| DDR2_v3p3_1p8v_bd\b17a_v5p0_1p8v_bd.ibs * IBIS 5.0 Model
| Die rev "A"
| 512Gb High Speed TLC Nand Flash IBIS Model
| VCC=2.7V-3.6V, VCCQ=1.7V-1.95V
| Temperature range, Commercial 0C to 70C.
| Part Number   VCC/VCCQ   Architecture  Mode   Package
| MT29F512G08EBCAFB17A  3.3/1.8V   512Gig x 8   NV-DDR2  Bare Die
[IBIS Ver]   5.0
[File name]   DDR2_v3p3_1p8v_bd.ibs
[Date]   01/31/2018
[File Rev]   2.0
[Source]   From silicon level SPICE model at Micron Technology, Inc.
   For support e-mail modelsupport@micron.com
[Notes]   Revision History:
   Rev 1.0: 12/12/2016
   - First revision pre-silicon model from parasitic extracted netlist
   Rev 2.0: 01/31/2018
   - Matched C_comp with latest IOCAP measurements
   - Matched IV curves with latest silicon measurements
   Notes:
   - This IBIS file uses the Submodel keyword to model the
   NV-DDR2 On-die Termination(ODT) characteristics.
   - The C_comp value in the DQ model is set to match the input
   state of the DQ I/O as measured from the HSpice model.
   Due to the C_comp differences between the DQ model and the
   DQ_ODT* models, the output characteristics of the
   models will look different when simulated. To match most
   closely with the HSPICE model, simulate with the
   DQ_35 or DQ_50 model for ALL Output simulations.
   Use the ODT models ONLY for Input simulations.
   - All Submodels: when running through ibischk4.2, this file
   contains warnings about GND and Power Clamp data being
   non-monotonic. When Submodel I-V curves are added to
   non-ODT Power and GND Clamp curves, the resultant
   curve is monotonic. This is not checked correctly with this
   version of the IBIS parser.
   - No Power Clamp Diode in models INPUT, CE_INPUT, WP_INPUT
   and RDBY
   - Typ and slow corner V-t curves in the DQ* models
   are shifted relative to strong corner V-t curve
   to contain all 3 corners within appropriate V-t window
   Models   Typ   Slow   V-t duration
   DQ_35_EXT_ZQ  -0.16ns   -0.39ns   2.38ns
   DQ_50_EXT_ZQ  -0.16ns   -0.39ns   2.38ns
   DQ_35_NO_ZQ   -0.16ns   -0.39ns   2.38ns
   DQ_50_NO_ZQ   -0.16ns   -0.39ns   2.38ns
   - Due to the shift in typ and slow corner, the V-t curves
   may overlap each other. This does not effect the accuracy
   of the IBIS data.
   - Model syntax should be checked using the latest IBISCHK parser,
   Version 6.1.2 or later.  Earlier versions may indicate erroneous
   Errors, Warnings or Cautions due to parser bugs.
   - All DQ/DQS models require overclocking due to inclusion of
   Composite Current data.
   - IBIS Quality Specification 2.0 Summary:
   IQ Score: IQ3MSX
   See Micron IBIS Model Quality Report and Quality Checklist
   for full IQ details
[Disclaimer]  This software code and all associated documentation, comments
   or other information (collectively "Software") is provided
   "AS IS" without warranty of any kind. MICRON TECHNOLOGY, INC.
   ("MTI") EXPRESSLY DISCLAIMS ALL WARRANTIES EXPRESS OR IMPLIED,
   INCLUDING BUT NOT LIMITED TO, NONINFRINGEMENT OF THIRD PARTY
   RIGHTS, AND ANY IMPLIED WARRANTIES OF MERCHANTABILITY OR
   FITNESS FOR ANY PARTICULAR PURPOSE. MTI DOES NOT WARRANT THAT
   THE SOFTWARE WILL MEET YOUR REQUIREMENTS, OR THAT THE
   OPERATION OF THE SOFTWARE WILL BE UNINTERRUPTED OR ERROR-FREE.
   FURTHERMORE, MTI DOES NOT MAKE ANY REPRESENTATIONS REGARDING
   THE USE OR THE RESULTS OF THE USE OF THE SOFTWARE IN TERMS OF
   ITS CORRECTNESS, ACCURACY, RELIABILITY, OR OTHERWISE. THE
   ENTIRE RISK ARISING OUT OF USE OR PERFORMANCE OF THE SOFTWARE
   REMAINS WITH YOU. IN NO EVENT SHALL MTI, ITS AFFILIATED
   COMPANIES OR THEIR SUPPLIERS BE LIABLE FOR ANY DIRECT,
   INDIRECT, CONSEQUENTIAL, INCIDENTAL, OR SPECIAL DAMAGES
   (INCLUDING, WITHOUT LIMITATION, DAMAGES FOR LOSS OF PROFITS,
   BUSINESS INTERRUPTION, OR LOSS OF INFORMATION) ARISING OUT OF
   YOUR USE OF OR INABILITY TO USE THE SOFTWARE, EVEN IF MTI HAS
   BEEN ADVISED OF THE POSSIBILITY OF SUCH DAMAGES. Because some
   jurisdictions prohibit the exclusion or limitation of
   liability for consequential or incidental damages, the above
   limitation may not apply to you.
[Copyright]   Copyright 2018 Micron Technology, Inc. All rights reserved.
|   COMPONENT: MT29F512G08EBCAFB17A
[Component]   MT29F512G08EBCAFB17A
[Manufacturer]  Micron Technology, Inc.
[Package]
| variable   typ   min   max
R_pkg   0.001m   0.001m   0.001m
L_pkg   0.001nH   0.001nH   0.001nH
C_pkg   0.001pf   0.001pf   0.001pf
[Pin]   signal_name model_name   R_pin   L_pin   C_pin
1   VSS   GND
2   VSS   GND
3   VCC   POWER
4   DNU   NC
5   MDS3   NC
6   MDS2   NC
7   MDS1   NC
8   MDS0   NC
9   Eno   NC
10   Eni   NC
11   WP#   WP_INPUT
12   DNU   NC
13   ALE   INPUT
14   CLE   INPUT
15   VSS   GND
16   VCC   POWER
17   VCCQ   POWER
18   DQ0   DQ
19   DQ1   DQ
20   VSSQ   GND
21   DQ2   DQ
22   DQ3   DQ
23   VCCQ   POWER
24   DQS_c   DQS
25   DQS_t   DQS
26   VSSQ   GND
27   DQ4   DQ
28   DQ5   DQ
29   VCCQ   POWER
30   DQ6   DQ
31   DQ7   DQ
32   VSSQ   GND
33   RE_c   RE
34   RE_t   RE
35   VCCQ   POWER
36   VCC   POWER
37   WE#   INPUT
38   DNU   NC
39   CE#   CE_INPUT
40   DNU   NC
41   RB#   RDBY
42   VCCQ   POWER
43   VREFQ   POWER
44   VSSQ   GND
45   ZQ   NC
46   VCCQ   POWER
47   VPP   POWER
48   DNU   NC
49   DNU   NC
50   VCC   POWER
|**********************DIFF PIN*********************************************
[Diff_pin]   inv_pin   vdiff   tdelay_typ   tdelay_min   tdelay_max
   25   24   0.300V   0ns   NA   NA
   34   33   0.300V   0ns   NA   NA
|   Model Selector
[Model Selector] DQ
DQ_35_EXT_ZQ   35 Ohm Data I/O with no ODT, With ZQ Cal
DQ_50_EXT_ZQ   50 Ohm Data I/O with no ODT, With ZQ Cal
DQ_IN_ODT50_EXT_ZQ   Data Input with 50ohm ODT, With ZQ Cal
DQ_IN_ODT75_EXT_ZQ   Data Input with 75ohm ODT, With ZQ Cal
DQ_IN_ODT100_EXT_ZQ   Data Input with 100ohm ODT, With ZQ Cal
DQ_IN_ODT150_EXT_ZQ   Data Input with 150ohm ODT, With ZQ Cal
DQ_25_NO_ZQ   25 Ohm Data I/O with no ODT, With No Cal
DQ_35_NO_ZQ   35 Ohm Data I/O with no ODT, With No Cal
DQ_50_NO_ZQ   50 Ohm Data I/O with no ODT, With No Cal
DQ_IN_ODT50_NO_ZQ   Data Input with 50ohm ODT, With No Cal
DQ_IN_ODT75_NO_ZQ   Data Input with 75ohm ODT, With No Cal
DQ_IN_ODT100_NO_ZQ   Data Input with 100ohm ODT, With No Cal
DQ_IN_ODT150_NO_ZQ   Data Input with 150ohm ODT, With No Cal
[Model Selector] DQS
DQS_35_EXT_ZQ   35 Ohm Data Strobe I/O with no ODT, With ZQ Cal
DQS_50_EXT_ZQ   50 Ohm Data Strobe I/O with no ODT, With ZQ Cal
DQS_IN_ODT50_EXT_ZQ   Data Strobe Input with 50ohm ODT, With ZQ Cal
DQS_IN_ODT75_EXT_ZQ   Data Strobe Input with 75ohm ODT, With ZQ Cal
DQS_IN_ODT100_EXT_ZQ   Data Strobe Input with 100ohm ODT, With ZQ Cal
DQS_IN_ODT150_EXT_ZQ   Data Strobe Input with 150ohm ODT, With ZQ Cal
DQS_25_NO_ZQ   25 Ohm Data Strobe I/O with no ODT, With No Cal
DQS_35_NO_ZQ   35 Ohm Data Strobe I/O with no ODT, With No Cal
DQS_50_NO_ZQ   50 Ohm Data Strobe I/O with no ODT, With No Cal
DQS_IN_ODT50_NO_ZQ   Data Strobe Input with 50ohm ODT, With No Cal
DQS_IN_ODT75_NO_ZQ   Data Strobe Input with 75ohm ODT, With No Cal
DQS_IN_ODT100_NO_ZQ   Data Strobe Input with 100ohm ODT, With No Cal
DQS_IN_ODT150_NO_ZQ   Data Strobe Input with 150ohm ODT, With No Cal
[Model Selector] RE
RE_INPUT   RE Input Model with no ODT
RE_INPUT_ODT50_EXT_ZQ   RE Input Model with 50ohm ODT, With ZQ Cal
RE_INPUT_ODT75_EXT_ZQ   RE Input Model with 75ohm ODT, With ZQ Cal
RE_INPUT_ODT100_EXT_ZQ  RE Input Model with 100ohm ODT, With ZQ Cal
RE_INPUT_ODT150_EXT_ZQ  RE Input Model with 150ohm ODT, With ZQ Cal
RE_INPUT_ODT50_NO_ZQ   RE Input Model with 50ohm ODT, With No Cal
RE_INPUT_ODT75_NO_ZQ   RE Input Model with 75ohm ODT, With No Cal
RE_INPUT_ODT100_NO_ZQ   RE Input Model with 100ohm ODT, With No Cal
RE_INPUT_ODT150_NO_ZQ   RE Input Model with 150ohm ODT, With No Cal
[Model Selector] RDBY
RDBY_FULL   FULL-Drv RDBY Open-Drain Model
RDBY_3QTR   3QTR-Drv RDBY Open-Drain Model
RDBY_HALF   HALF-Drv RDBY Open-Drain Model
RDBY_QTR   QTR-Drv RDBY Open-Drain Model
| Models and submodels in the file (50): DQ_35_EXT_ZQ (I/O), DQ_50_EXT_ZQ (I/O), DQ_IN_ODT50_EXT_ZQ (Input), DQ_IN_ODT75_EXT_ZQ (Input), DQ_IN_ODT100_EXT_ZQ (Input), DQ_IN_ODT150_EXT_ZQ (Input), DQ_25_NO_ZQ (I/O), DQ_35_NO_ZQ (I/O), DQ_50_NO_ZQ (I/O), DQ_IN_ODT50_NO_ZQ (Input), DQ_IN_ODT75_NO_ZQ (Input), DQ_IN_ODT100_NO_ZQ (Input), DQ_IN_ODT150_NO_ZQ (Input), DQS_35_EXT_ZQ (I/O), DQS_50_EXT_ZQ (I/O), DQS_IN_ODT50_EXT_ZQ (Input), DQS_IN_ODT75_EXT_ZQ (Input), DQS_IN_ODT100_EXT_ZQ (Input), DQS_IN_ODT150_EXT_ZQ (Input), DQS_25_NO_ZQ (I/O), DQS_35_NO_ZQ (I/O), DQS_50_NO_ZQ (I/O), DQS_IN_ODT50_NO_ZQ (Input), DQS_IN_ODT75_NO_ZQ (Input), DQS_IN_ODT100_NO_ZQ (Input), DQS_IN_ODT150_NO_ZQ (Input), INPUT (Input), CE_INPUT (Input), WP_INPUT (Input), RE_INPUT (Input), RE_INPUT_ODT50_EXT_ZQ (Input), RE_INPUT_ODT75_EXT_ZQ (Input), RE_INPUT_ODT100_EXT_ZQ (Input), RE_INPUT_ODT150_EXT_ZQ (Input), RE_INPUT_ODT50_NO_ZQ (Input), RE_INPUT_ODT75_NO_ZQ (Input), RE_INPUT_ODT100_NO_ZQ (Input), RE_INPUT_ODT150_NO_ZQ (Input), RDBY_FULL (Open_drain), RDBY_3QTR (Open_drain), RDBY_HALF (Open_drain), RDBY_QTR (Open_drain), 50ohm_ODT_EXT_ZQ (Dynamic_clamp), 75ohm_ODT_EXT_ZQ (Dynamic_clamp), 100ohm_ODT_EXT_ZQ (Dynamic_clamp), 150ohm_ODT_EXT_ZQ (Dynamic_clamp), 50ohm_ODT_NO_ZQ (Dynamic_clamp), 75ohm_ODT_NO_ZQ (Dynamic_clamp), 100ohm_ODT_NO_ZQ (Dynamic_clamp), 150ohm_ODT_NO_ZQ (Dynamic_clamp)
